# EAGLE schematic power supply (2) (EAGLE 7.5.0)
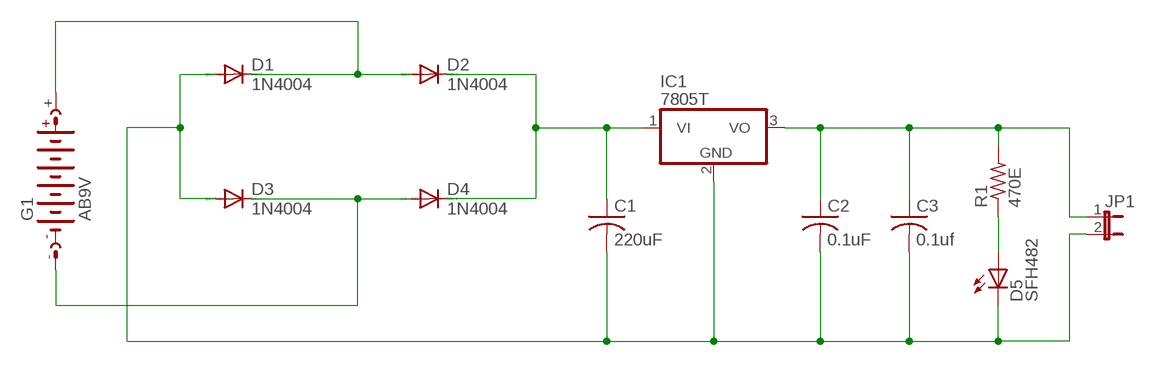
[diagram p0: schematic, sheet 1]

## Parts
C1  220uF  C-US050-030X075  [C050-030X075]
C2  0.1uF  C-US050-030X075  [C050-030X075]
C3  0.1uf  C-US050-030X075  [C050-030X075]
D1  1N4004  [DO41-10]
D2  1N4004  [DO41-10]
D3  1N4004  [DO41-10]
D4  1N4004  [DO41-10]
D5  SFH482  [SFH482]
G1  AB9V  [AB9V]
IC1  7805T  [TO220H]
JP1  JP1E  [JP1]
R1  470E  R-US_0204/7  [0204/7]

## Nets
N$1: C1.2 C2.2 C3.2 D1.A D3.A D5.K(C) IC1.2(GND) JP1.2
N$2: D1.C D2.A G1.+
N$3: C1.1 D2.C D4.C IC1.1(VI)
N$4: D3.C D4.A G1.-
N$7: C2.1 C3.1 IC1.3(VO) JP1.1 R1.2
N$8: D5.A R1.1

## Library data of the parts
C1-C3 = rcl:C-US: CAPACITOR, American symbol
D1-D4 = diode:1N4004: DIODE
D5 = led:SFH482: IR LED
G1 = battery:AB9V: 9-V BATTERY CLIP
IC1 = linear:78*: Positive VOLTAGE REGULATOR Source: http://cache.national.com/ds/LM/LM78L05.pdf http://www.fairchildsemi.com/ds/LM/LM7805.pdf
JP1 = jumper:JP1E: JUMPER
R1 = rcl:R-US_: RESISTOR, American symbol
